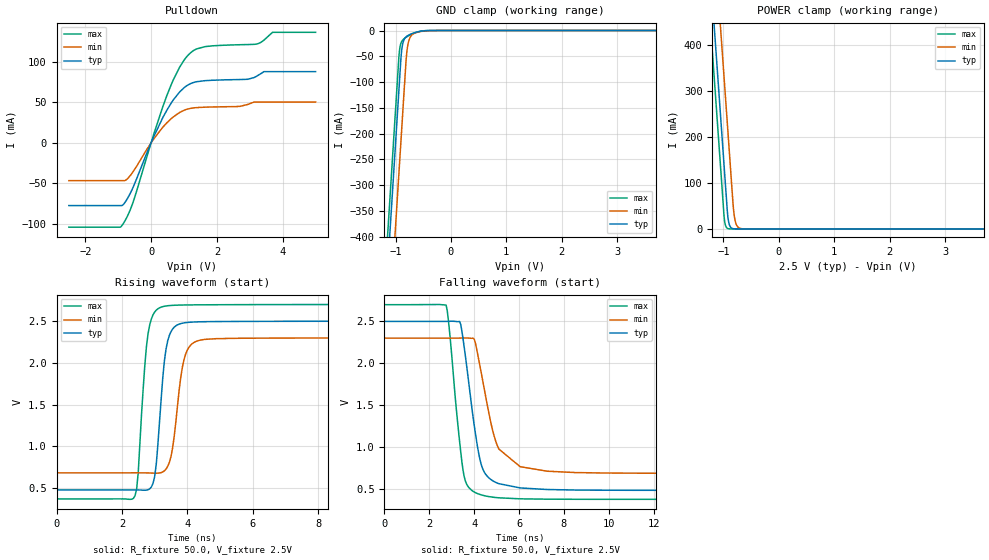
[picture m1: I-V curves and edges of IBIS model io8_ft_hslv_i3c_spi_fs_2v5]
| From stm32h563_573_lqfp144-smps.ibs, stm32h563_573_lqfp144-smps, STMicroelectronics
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[Model]   io8_ft_hslv_i3c_spi_fs_2v5
Model_type I/O_open_drain
Polarity   Non-Inverting
Enable   Active-Low
| CAP_THRESHOLD on pad IOFT is "UDTCAPC" :
| Rising=20.0% of vddiom   Falling=80.0% of vddiom
| C_comp min and max val. don't necessarily correlate with the min and max pvt
| but are the smallest and greatest pad capacitance found.
| var   typ   min   max
C_comp   3.87733pF  3.87281pF  3.96699pF
|C_comp_pulldown   3.87733pF  3.87281pF  3.96699pF
Vinl = 1.15V
Vinh = 1.35V
Vmeas = 1.25V   | Reference voltage for timing measurements
Cref  = 50.0pF   | Timing specification test load capacitance value
Rref  = 1.0MOhm   | Timing specification test load resistance value
Vref  = 1.375V   | Timing specification test load voltage
[Model Spec]
| TIME_THRESHOLD on pin ZII2CV11 is "CMOS" :
| Rising=40.0% of vdd   Falling=60.0% of vdd
Vinl 989.80000mV 917.80000mV 1.06580V
Vinh 1.40320V 1.29620V 1.49120V
| variable   typ   min   max
[Temperature Range] 25.0 125.0 -40.0
| variable   typ   min   max
[Voltage Range] 2.5V 2.3V 2.7V
| variable   typ   min   max
[POWER Clamp Reference] 2.5V 2.3V 2.7V
| variable   typ   min   max
[GND Clamp Reference] 0V 0V 0V
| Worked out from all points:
|   slope of the pulldown table from 0 to 0.375 V, typ, clamps not added: 11.5 ohm
|   GND clamp passes 1 mA (typ) near -0.52 V on its own axis
|   POWER clamp passes 1 mA (typ) near -0.84 V on its own axis
|   rising waveform, R_fixture 50.0, V_fixture 2.5V: 20-80 % time 254ps typ, 305ps min, 242ps max; typ from 0.481 V to 2.5 V
|   falling waveform, R_fixture 50.0, V_fixture 2.5V: 20-80 % time 627ps typ, 794ps min, 492ps max; typ from 2.5 V to 0.481 V
[POWER Clamp]
-2.5V     2.708A     2.899A     2.597A
-1.23V    548.8mA    740.2mA    437.5mA
-1.16V    429.8mA    621.2mA    318.5mA
-1.12V    361.8mA    553.2mA    250.5mA
-1.03V    208.8mA    400.2mA    97.53mA
-980mV    123.8mA    315.2mA    17.95mA
-920mV    26.3mA     213.2mA    906uA
-880mV    5.543mA    145.2mA    123.7uA
-810mV    363.5uA    33.6mA     3.797uA
-770mV    76.62uA    10.47mA    518.8nA
-700mV    5.026uA    1.361mA    16.11nA
5V        0A         0A         0A
[GND Clamp]
-2.5V     -2.77A     -2.931A    -2.704A
-1.21V    -576.8mA   -738.1mA   -511.3mA
-950mV    -134.8mA   -296.1mA   -69.34mA
-920mV    -83.82mA   -245.1mA   -32.48mA
-900mV    -50.56mA   -211.1mA   -24.02mA
-880mV    -31.31mA   -177.1mA   -19.85mA
-850mV    -18.7mA    -126.1mA   -16.34mA
-800mV    -11.46mA   -46.18mA   -12.45mA
-750mV    -8.203mA   -16.63mA   -9.325mA
-650mV    -4.063mA   -4.987mA   -4.427mA
-360mV    -35.05uA   -165.1uA   -9.564uA
5V        7.96nA     1.281uA    294pA
| variable   typ   min   max
[Pullup Reference] 2.5V 2.3V 2.7V
| variable   typ   min   max
[Pulldown Reference] 0V 0V 0V
[Pulldown]
-2.5V     -77.63mA   -46.85mA   -104.3mA
-870mV    -77.24mA   -46.85mA   -101.4mA
-550mV    -55.3mA    -35.88mA   -73.72mA
90mV      8.401mA    5.299mA    11.79mA
610mV     49.03mA    29.76mA    71.69mA
870mV     62.92mA    37.48mA    93.62mA
1.23V     73.63mA    42.72mA    112.2mA
1.64V     76.78mA    44.01mA    118.8mA
2.7V      78.15mA    44.99mA    121.2mA
3.22V     82.58mA    50.35mA    122.2mA
3.69V     87.93mA    50.35mA    136.5mA
5V        87.93mA    50.35mA    136.5mA
[Ramp]
dV/dt_r 1.21162V/249.73161ps 969.22782mV/302.5337ps 1.39626V/238.7174ps
dV/dt_f 1.21165V/625.53493ps 969.26173mV/793.85655ps 1.39628V/491.53323ps
R_load = 50.0
| Removed startup time: 0s 0s 0s  .
| Removed end time: 34.4ns.
[Rising Waveform]
R_fixture   = 50.0
V_fixture   = 2.5V
V_fixture_min = 2.3V
V_fixture_max = 2.7V
0s        480.6mV    684.6mV    372.9mV
2.4ns     480.4mV    684.8mV    409.6mV
2.5ns     480.1mV    684.7mV    696.2mV
2.8ns     482.1mV    683.6mV    2.352V
3.05ns    787.5mV    680.3mV    2.632V
3.35ns    2.169V     730.3mV    2.682V
3.55ns    2.406V     982.4mV    2.69V
3.9ns     2.48V      2.042V     2.694V
4.5ns     2.494V     2.28V      2.696V
34.4ns    2.5V       2.3V       2.7V
| Removed startup time: 0s 0s 0s  .
| Removed end time: 59.35ns.
[Falling Waveform]
R_fixture   = 50.0
V_fixture   = 2.5V
V_fixture_min = 2.3V
V_fixture_max = 2.7V
0s        2.5V       2.3V       2.7V
2.75ns    2.5V       2.3V       2.695V
3.35ns    2.5V       2.3V       1.067V
3.6ns     2.105V     2.302V     599.2mV
4ns       1.263V     2.288V     461mV
4.35ns    760.6mV    1.836V     423.6mV
4.75ns    608.7mV    1.282V     401.6mV
6.05ns    509mV      763.3mV    378.9mV
8.5ns     484mV      693.1mV    373.4mV
59.35ns   480.6mV    684.6mV    372.9mV
